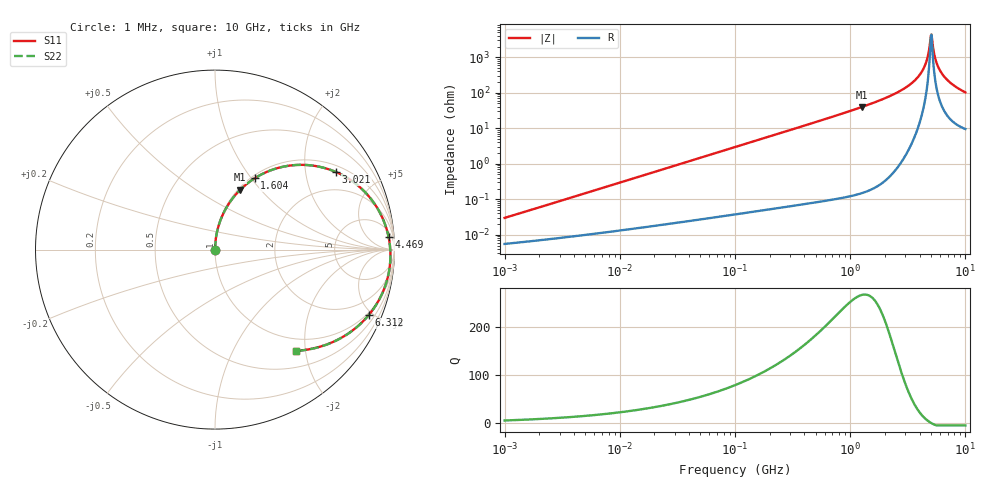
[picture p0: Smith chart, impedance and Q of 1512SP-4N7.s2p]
# MHz  S  MA  R  50
!Freq  MagS11  AngS11  MagS21  AngS21  MagS12  AngS12  MagS22  AngS22
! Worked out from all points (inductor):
!   801 points, 1 MHz to 10 GHz, reference 50 ohm
!   read as one part in series: L = 4.69 nH near 1.047 MHz
!   highest Q = 266 at 1.274 GHz (marker M1), where L = 5.01 nH
!   self-resonance near 5.014 GHz
!   S11 on the Smith chart (normalised r, x): 1 MHz: 1.00, +0.00; 1.604 GHz: 1.04, +1.04; 3.021 GHz: 1.22, +2.95; 4.469 GHz: 10, +23; 6.312 GHz: 0.87, -4.74; 10 GHz: 0.77, -1.82
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1  0.0002905 79.0  0.9999 -0.0  0.9999 -0.0  0.0002905 79.0
4.67769  0.001337 85.8  0.9999 -0.1  0.9999 -0.1  0.001337 85.8
21.6303  0.00617 87.9  0.9998 -0.4  0.9998 -0.4  0.00617 87.9
100.0216  0.02851 87.5  0.9992 -1.7  0.9992 -1.7  0.02851 87.5
467.8699  0.1333 81.5  0.9903 -8.2  0.9903 -8.2  0.1333 81.5
832.0259  0.2369 75.1  0.9705 -14.6  0.9705 -14.6  0.2369 75.1
1273.93  0.362 67.1  0.9308 -22.6  0.9308 -22.6  0.3619 67.1
1603.8  0.454 61.0  0.8892 -28.8  0.8892 -28.8  0.4539 61.0
2163.497  0.6039 50.1  0.7939 -39.6  0.7939 -39.6  0.6037 50.1
3021.086  0.8005 32.7  0.5893 -56.6  0.5893 -56.6  0.8004 32.7
3847.406  0.9253 16.0  0.3474 -72.0  0.3474 -72.0  0.9252 16.0
4170.322  0.9534 9.7  0.2501 -76.9  0.2501 -76.9  0.9534 9.7
4468.595  0.9697 4.2  0.1626 -79.7  0.1626 -79.7  0.9696 4.2
4679.204  0.976 0.5  0.1034 -79.0  0.1034 -79.0  0.976 0.5
4899.739  0.9785 -3.2  0.04606 -66.7  0.04606 -66.7  0.9786 -3.2
5071.934  0.978 -6.0  0.02231 4.2  0.02231 4.2  0.978 -6.0
5250.182  0.9754 -8.8  0.05408 55.6  0.05408 55.6  0.9755 -8.8
5497.627  0.9689 -12.5  0.1104 64.3  0.1104 64.3  0.969 -12.5
5690.835  0.9618 -15.2  0.1528 64.7  0.1528 64.7  0.9619 -15.2
6312.161  0.9308 -23.1  0.2735 60.3  0.2735 60.3  0.9311 -23.1
7676.832  0.8465 -36.5  0.4627 48.4  0.4627 48.4  0.847 -36.5
10000  0.7218 -51.4  0.6331 33.7  0.6331 33.7  0.7229 -51.5
